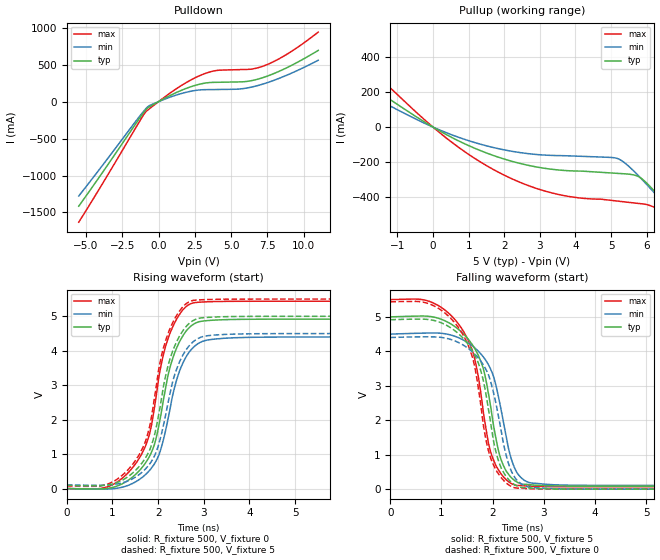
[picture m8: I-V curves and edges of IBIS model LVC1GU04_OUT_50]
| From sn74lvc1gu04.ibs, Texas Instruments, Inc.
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[Model]   LVC1GU04_OUT_50
Model_type  Output
Vref =   0
Rref =   500
Cref =   50p
Vmeas =   2.5
| variable   typ   min   max
C_comp   9.34pF   3.27pF   15.59pF
| C_pullup   11.19pF   4.59pF   15.59pF
| C_pulldown   7.50pF   3.27pF   12.02pF
[Temperature Range]   40   100   -40
| Ambient temperature   25   85   -40
[Voltage range]   5   4.5   5.5
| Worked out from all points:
|   slope of the pulldown table from 0 to 0.75 V, typ, clamps not added: 9.58 ohm
|   slope of the pullup table from 0 to 0.75 V, typ, clamps not added: 9.16 ohm
|   rising waveform, R_fixture 500, V_fixture 0: 20-80 % time 531ps typ, 518ps min, 545ps max; typ from 0 V to 4.92 V
|   falling waveform, R_fixture 500, V_fixture 5: 20-80 % time 449ps typ, 429ps min, 457ps max; typ from 5 V to 0.09 V
|   rising waveform, R_fixture 500, V_fixture 5: 20-80 % time 529ps typ, 517ps min, 541ps max; typ from 0.09 V to 5 V
|   falling waveform, R_fixture 500, V_fixture 0: 20-80 % time 447ps typ, 431ps min, 456ps max; typ from 4.92 V to 0 V
[Pulldown]
| LVC1GU04_OUT_50
|   Voltage   I(typ)   I(min)   I(max)
-5.5V     -1.415A    -1.277A    -1.632A
-3.76V    -929mA     -835.6mA   -1.077A
-1.165V   -184.5mA   -162.9mA   -220.2mA
-735mV    -83.52mA   -68.69mA   -112.1mA
1.09V     110.8mA    80.82mA    156.5mA
2.725V    230.9mA    156.2mA    342.2mA
3.95V     261.4mA    164mA      420mA
5.98V     271.4mA    181.1mA    435.5mA
6.58V     291.6mA    204.9mA    446.2mA
7.255V    329.4mA    241.9mA    484.3mA
8.925V    467.7mA    365.4mA    651.4mA
11V       693.7mA    560.3mA    941.4mA
[Pullup]
| LVC1GU04_OUT_50
|   Voltage   I(typ)   I(min)   I(max)
-5.5V     783.3mA    622.7mA    1.091A
-4.25V    594.9mA    469.5mA    833.1mA
-3.135V   430.4mA    337mA      606.3mA
580mV     -64.72mA   -47.9mA    -94.8mA
1.695V    -162.1mA   -116.6mA   -242.3mA
2.855V    -225.8mA   -155.4mA   -347.2mA
5.235V    -265.1mA   -184.2mA   -424mA
5.885V    -298.4mA   -302.4mA   -439mA
6.375V    -402.3mA   -411.7mA   -474mA
6.825V    -511.2mA   -516.1mA   -577.8mA
7.16V     -595mA     -595.3mA   -668.4mA
11V       -1.603A    -1.534A    -1.792A
[Ramp]
| LVC1GU04_OUT_50
| variable   typ   min   max
dV/dt_r   2.96/5.40E-10   2.65/5.25E-10   3.27/5.52E-10
dV/dt_f   2.96/4.62E-10   2.66/4.46E-10   3.27/4.71E-10
R_load = 500
[Rising Waveform]
| LVC1GU04_OUT_50
R_fixture =   500
C_fixture =   0
L_fixture =   0
V_fixture =   0
V_fixture_min = 0
V_fixture_max = 0
|   Time   V(typ)   V(min)   V(max)
0s        48.17pV    4.011nV    1.536nV
985ps     25.79mV    -7.798mV   99.34mV
1.66ns    627.9mV    332mV      1.051V
1.815ns   941.4mV    528.9mV    1.592V
1.93ns    1.323V     738.4mV    2.431V
2.075ns   2.241V     1.208V     3.64V
2.25ns    3.461V     2.229V     4.468V
2.52ns    4.381V     3.573V     5.148V
2.885ns   4.837V     4.215V     5.408V
50ns      4.917V     4.401V     5.437V
[Falling Waveform]
| LVC1GU04_OUT_50
R_fixture =   500
C_fixture =   0
L_fixture =   0
V_fixture =   5
V_fixture_min = 4.5
V_fixture_max = 5.5
|   Time   V(typ)   V(min)   V(max)
0s        5V         4.5V       5.5V
1.175ns   4.802V     4.477V     5.058V
1.55ns    4.301V     4.217V     4.226V
1.75ns    3.779V     3.957V     2.985V
1.99ns    2.119V     3.379V     950.3mV
2.18ns    794.6mV    2.194V     414.9mV
2.335ns   385.1mV    1.035V     191.6mV
2.485ns   198.8mV    458mV      108.2mV
3.87ns    90.19mV    110.1mV    71.44mV
50ns      89.62mV    107.6mV    71.33mV
[Rising Waveform]
| LVC1GU04_OUT_50
R_fixture =   500
C_fixture =   0
L_fixture =   0
V_fixture =   5
V_fixture_min = 4.5
V_fixture_max = 5.5
|   Time   V(typ)   V(min)   V(max)
0s        89.62mV    107.6mV    71.33mV
970ps     120.8mV    109.8mV    169.3mV
1.63ns    711.1mV    452.2mV    1.09V
1.795ns   1.061V     677.4mV    1.694V
1.915ns   1.518V     925.7mV    2.585V
2.045ns   2.383V     1.43V      3.673V
2.19ns    3.414V     2.297V     4.393V
2.45ns    4.376V     3.615V     5.117V
2.81ns    4.905V     4.302V     5.469V
50ns      5V         4.5V       5.5V
[Falling Waveform]
| LVC1GU04_OUT_50
R_fixture =   500
C_fixture =   0
L_fixture =   0
V_fixture =   0
V_fixture_min = 0
V_fixture_max = 0
|   Time   V(typ)   V(min)   V(max)
0s        4.917V     4.401V     5.437V
1.13ns    4.73V      4.367V     5.031V
1.52ns    4.204V     4.087V     4.184V
1.705ns   3.716V     3.833V     3.084V
1.84ns    2.994V     3.553V     1.671V
1.97ns    1.843V     3.076V     864mV
2.16ns    640mV      1.751V     347.9mV
2.305ns   295.1mV    769mV      133.6mV
2.475ns   92.19mV    258.3mV    31.36mV
50ns      3.012nV    4.499nV    3.558nV
